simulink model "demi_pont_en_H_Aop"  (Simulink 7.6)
settings: Solver=ode15s  StartTime=0.0  StopTime=0.8  RelTol=1e-3
InitFcn:
  | clc
  | delete *.mat
StopFcn:
  | close all, clc
  | load demi_pont_en_H_Aop.mat
  | [AX,H1,H2] = plotyy(x(1,:),x(2,:),x(1,:),x(3,:),'plot');
  | set(get(AX(1),'Ylabel'),'String','Vitesse angulaire')
  | set(get(AX(2),'Ylabel'),'String','Position angulaire')
  | xlabel('temps')
  | title('Position et vitesse angulaires - Moteur CC, 1/2 Pont en H')
  | grid
  | %axis([0 N -0.2 1.2])
undefined symbols (not defined in the file or in its folder): sigbuilder_block
libraries: elec_lib x9, fl_lib x8, nesl_utility x4

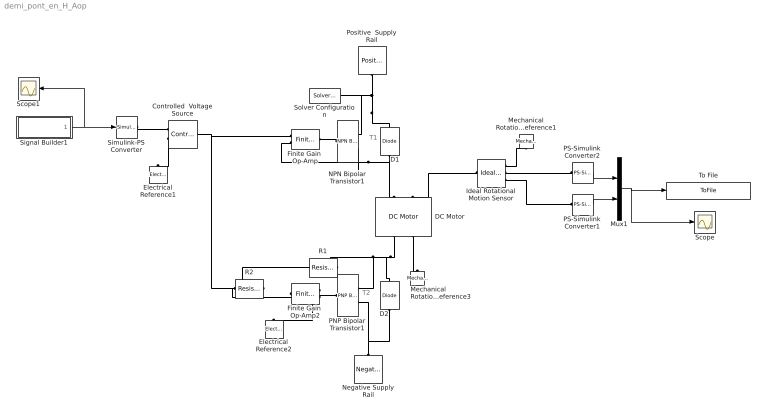
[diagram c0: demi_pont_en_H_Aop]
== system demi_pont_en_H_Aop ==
  note: T1
  note: T2
  Controlled  Voltage Source : fl_lib/Electrical/Electrical Sources/Controlled Voltage Source  DialogController=NetworkEngine.DynNeDlgSource  SystemSampleTime=-1  i_Log=off  v_Log=off  LocalVarNames=|i|v  LocalVarDescs=|i|v  LocalVarLogging=[0 0]
  D1 : elec_lib/Semiconductor Devices/Diode  DialogController=NetworkEngine.DynNeDlgSource  SystemSampleTime=-1  ModelType=1  Vf=0.6 V  Ron=0.3 Ohm  Goff=1e-8 S  Rz=0.3 Ohm  Vz=50 V  C_PWL=5 pF  prmExp=1  I12=[ 0.07 1.5 ] A  V12=[ 0.7 0.8 ] V  I1=0.07 A  V1=0.7 V  RS=0.01 Ohm  IS=1e-14 A  Tmeas=25 C  ec=1  BV=Inf V  C_param=1  CJ0=5 pF  VJ=1 V  Mgrad=0.5  Vvec=[ 0.1 10 100 ] V  Cvec=[ 3.5 1 0.4 ] pF  FC=0.5  LocalVarLogging=[]
  D2 : elec_lib/Semiconductor Devices/Diode  DialogController=NetworkEngine.DynNeDlgSource  SystemSampleTime=-1  ModelType=1  Vf=0.6 V  Ron=0.3 Ohm  Goff=1e-8 S  Rz=0.3 Ohm  Vz=50 V  C_PWL=5 pF  prmExp=1  I12=[ 0.07 1.5 ] A  V12=[ 0.7 0.8 ] V  I1=0.07 A  V1=0.7 V  RS=0.01 Ohm  IS=1e-14 A  Tmeas=25 C  ec=1  BV=Inf V  C_param=1  CJ0=5 pF  VJ=1 V  Mgrad=0.5  Vvec=[ 0.1 10 100 ] V  Cvec=[ 3.5 1 0.4 ] pF  FC=0.5  LocalVarLogging=[]
  DC Motor : elec_lib/Actuators & Drivers/Rotational Actuators/DC Motor  DialogController=NetworkEngine.DynNeDlgSource  SystemSampleTime=-1  parameterization=1  Ra=3.9 Ohm  La=1.2e-5 H  emf_or_torque=1  Kv=7.2e-5 V/rpm  Ki=6.876e-4 N*m/A  T_stall=2.4e-4 N*m  w_max=1.91e+4 rpm  w_rated=1.5e+4 rpm  P_rated=0.08 W  V_rated=1.5 V  J=0.01 g*cm^2  lam=1e-8 N*m/(rad/s)  speed0=0.5 rpm  current_Log=off  voltage_Log=off  power_Log=off  i2r_Log=off  torque_Log=off  speed_Log=off  LocalVarNames=|current|voltage|power|i2r|torque|speed  LocalVarDescs=|Current (A)|Voltage (V)|Power (W)|Electrical losses (W)|Torque (Nm)|Angular speed (rad/s)  LocalVarLogging=[0 0 0 0 0 0]
  Electrical Reference1 : fl_lib/Electrical/Electrical Elements/Electrical Reference  DialogController=NetworkEngine.DynNeDlgSource  SystemSampleTime=-1  i_Log=off  LocalVarNames=|i  LocalVarDescs=|i  LocalVarLogging=[]
  Electrical Reference2 : fl_lib/Electrical/Electrical Elements/Electrical Reference  DialogController=NetworkEngine.DynNeDlgSource  SystemSampleTime=-1  i_Log=off  LocalVarNames=|i  LocalVarDescs=|i  LocalVarLogging=[]
  Finite Gain  Op-Amp : elec_lib/Integrated Circuits/Finite Gain Op-Amp  DialogController=NetworkEngine.DynNeDlgSource  SystemSampleTime=-1  A=1000  Rin=1e+6 Ohm  Rout=100 Ohm  Vmin=-15 V  Vmax=15 V  LocalVarLogging=[]
  Finite Gain  Op-Amp2 : elec_lib/Integrated Circuits/Finite Gain Op-Amp  DialogController=NetworkEngine.DynNeDlgSource  SystemSampleTime=-1  A=1000  Rin=1e+6 Ohm  Rout=100 Ohm  Vmin=-15 V  Vmax=15 V  LocalVarLogging=[]
  Ideal Rotational Motion Sensor : fl_lib/Mechanical/Mechanical Sensors/Ideal Rotational Motion Sensor  DialogController=NetworkEngine.DynNeDlgSource  SystemSampleTime=-1  offset=0 rad  w_Log=off  t_Log=off  phi_Log=off  LocalVarNames=|w|t|phi  LocalVarDescs=|w|t|phi  LocalVarLogging=[0 0 0]
  Mechanical Rotational Reference1 : fl_lib/Mechanical/Rotational Elements/Mechanical Rotational Reference  DialogController=NetworkEngine.DynNeDlgSource  SystemSampleTime=-1  t_Log=off  LocalVarNames=|t  LocalVarDescs=|t  LocalVarLogging=0
  Mechanical Rotational Reference3 : fl_lib/Mechanical/Rotational Elements/Mechanical Rotational Reference  DialogController=NetworkEngine.DynNeDlgSource  SystemSampleTime=-1  t_Log=off  LocalVarNames=|t  LocalVarDescs=|t  LocalVarLogging=0
  Mux1 : Mux  Inputs=2
  NPN Bipolar Transistor1 : elec_lib/Semiconductor Devices/NPN Bipolar Transistor  DialogController=NetworkEngine.DynNeDlgSource  SystemSampleTime=-1  parameterization=1  BF=100  IS=1e-14 A  VAF=200 V  hfe=100  hoe=5e-5 1/Ohm  Ic_h=1 mA  V1=0.55 V  I1=0.5 mA  BR=1  Tmeas=25 C  RC=0.01 Ohm  RE=1e-4 Ohm  RB=1 Ohm  C_BC=5 pF  C_BE=5 pF  TF=0 us  TR=0 us  LocalVarLogging=[]
  Negative Supply Rail : elec_lib/Sources/Negative Supply Rail  DialogController=NetworkEngine.DynNeDlgSource  SystemSampleTime=-1  v0=-24 V  current_Log=off  voltage_Log=off  power_Log=off  LocalVarNames=|current|voltage|power  LocalVarDescs=|Current (A)|Voltage (V)|Power (W)  LocalVarLogging=[0 0 0]
  PNP Bipolar Transistor1 : elec_lib/Semiconductor Devices/PNP Bipolar Transistor  DialogController=NetworkEngine.DynNeDlgSource  SystemSampleTime=-1  parameterization=1  BF=100  IS=1e-14 A  VAF=200 V  hfe=100  hoe=5e-5 1/Ohm  Ic_h=1 mA  V1=0.55 V  I1=0.5 mA  BR=1  Tmeas=25 C  RC=0.01 Ohm  RE=1e-4 Ohm  RB=1 Ohm  C_BC=5 pF  C_BE=5 pF  TF=0 us  TR=0 us  LocalVarLogging=[]
  PS-Simulink Converter1 : nesl_utility/PS-Simulink Converter  DialogController=NetworkEngine.DynNeUtilDlgSource  SystemSampleTime=-1  PhysicalDomain=network_engine_domain  LeftPortType=input  RightPortType=output  SubClassName=ps_output  Unit=1  AffineConversion=off
  PS-Simulink Converter2 : nesl_utility/PS-Simulink Converter  DialogController=NetworkEngine.DynNeUtilDlgSource  SystemSampleTime=-1  PhysicalDomain=network_engine_domain  LeftPortType=input  RightPortType=output  SubClassName=ps_output  Unit=1  AffineConversion=off
  Positive  Supply Rail : elec_lib/Sources/Positive Supply Rail  DialogController=NetworkEngine.DynNeDlgSource  SystemSampleTime=-1  v0=24 V  current_Log=off  voltage_Log=off  power_Log=off  LocalVarNames=|current|voltage|power  LocalVarDescs=|Current (A)|Voltage (V)|Power (W)  LocalVarLogging=[0 0 0]
  R1 : fl_lib/Electrical/Electrical Elements/Resistor  DialogController=NetworkEngine.DynNeDlgSource  SystemSampleTime=-1  R=10 kOhm  i_Log=off  v_Log=off  LocalVarNames=|i|v  LocalVarDescs=|i|v  LocalVarLogging=[0 0]
  R2 : fl_lib/Electrical/Electrical Elements/Resistor  DialogController=NetworkEngine.DynNeDlgSource  SystemSampleTime=-1  R=10 kOhm  i_Log=off  v_Log=off  LocalVarNames=|i|v  LocalVarDescs=|i|v  LocalVarLogging=[0 0]
  Scope : Scope
  Scope1 : Scope
  Signal Builder1 : Subsystem  Tag=STV Subsys  LoadFcn=sigbuilder_block('load');  StartFcn=sigbuilder_block('start');  StopFcn=sigbuilder_block('stop');  ClipboardFcn=sigbuilder_block('clipboard');
  Simulink-PS Converter : nesl_utility/Simulink-PS Converter  DialogController=NetworkEngine.DynNeUtilDlgSource  SystemSampleTime=-1  PhysicalDomain=network_engine_domain  LeftPortType=input  RightPortType=output  SubClassName=ps_input  Unit=1  AffineConversion=off  InputFilterTimeConstant=.001  UdotUserProvided=0
  Solver Configuration : nesl_utility/Solver Configuration  DialogController=NetworkEngine.DynNeUtilDlgSource  SystemSampleTime=-1  PhysicalDomain=network_engine_domain  LeftPortType=input  RightPortType=generic  SubClassName=solver  Accelerate=off  Profile=off  ResidualTolerance=1e-9  MaxNonlinIter=3  MaxModeIter=2  DoFixedCost=off  UseLocalSampling=off  DoDC=off  LinearAlgebra=Sparse  LocalSolverSampleTime=.001  LocalSolverChoice=NE_BACKWARD_EULER_ADVANCER  UseLocalSolver=off
  To File : ToFile  Filename=demi_pont_en_H_Aop  MatrixName=x
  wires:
  Signal Builder1/1(Signal 1) -> Simulink-PS Converter/1, Scope1/1
  PS-Simulink Converter1/1 -> Mux1/2
  PS-Simulink Converter2/1 -> Mux1/1
  Mux1/1 -> Scope/1, To File/1
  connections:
  NPN Bipolar Transistor1/LConn1 -- Finite Gain  Op-Amp/RConn1
  NPN Bipolar Transistor1/RConn1 -- D1/RConn1 -- Positive  Supply Rail/RConn1 -- Solver Configuration/RConn1
  Simulink-PS Converter/RConn1 -- Controlled  Voltage Source/RConn1
  D1/LConn1 -- Finite Gain  Op-Amp/LConn2 -- NPN Bipolar Transistor1/RConn2 -- DC Motor/LConn1
  DC Motor/RConn1 -- R1/RConn1 -- PNP Bipolar Transistor1/RConn1 -- D2/RConn1
  Negative Supply Rail/LConn1 -- PNP Bipolar Transistor1/RConn2 -- D2/LConn1
  DC Motor/RConn2 -- Mechanical Rotational Reference3/LConn1
  Ideal Rotational Motion Sensor/LConn1 -- DC Motor/LConn2
  Finite Gain  Op-Amp2/RConn1 -- PNP Bipolar Transistor1/LConn1
  R2/RConn1 -- Finite Gain  Op-Amp2/LConn2 -- R1/LConn1
  Finite Gain  Op-Amp2/LConn1 -- Electrical Reference2/LConn1
  Controlled  Voltage Source/RConn2 -- Electrical Reference1/LConn1
  Ideal Rotational Motion Sensor/RConn3 -- PS-Simulink Converter1/LConn1
  Ideal Rotational Motion Sensor/RConn2 -- PS-Simulink Converter2/LConn1
  Ideal Rotational Motion Sensor/RConn1 -- Mechanical Rotational Reference1/LConn1
  Controlled  Voltage Source/LConn1 -- Finite Gain  Op-Amp/LConn1 -- R2/LConn1

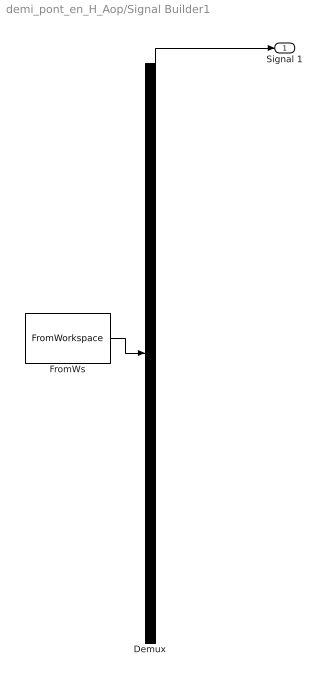
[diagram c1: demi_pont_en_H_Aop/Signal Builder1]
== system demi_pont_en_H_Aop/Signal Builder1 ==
  Demux : Demux  Tag=STV Demux  Outputs=1
  FromWs : FromWorkspace  Tag=STV FromWs  VariableName=tuvar  SampleTime=0  SigBuilderData=DataTag0  VnvData=DataTag1
  Signal 1 : Outport  Tag=STV Outport
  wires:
  FromWs/1 -> Demux/1
  Demux/1 -> Signal 1/1
